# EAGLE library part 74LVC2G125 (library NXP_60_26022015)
Dual bus buffer/line driver; 3-state The 74LVC2G125 provides a dual non-inverting buffer/line driver with 3-state output. The 3-state output is controlled by the output enable input (pin nOE). A HIGH-level at pin nOE causes the output to assume a high-impedance OFF-state. Schmitt trigger action at all inputs makes the circuit highly tolerant of slower input rise and fall times. Inputs can be driven from either 3.3 V or 5 V devices. This feature allows the use of these devices as translators in a mixed 3.3 V and 5 V environment. This device is fully specified for partial power-down applications using IOFF. The IOFF circuitry disables the output, preventing a damaging backflow current through the device when it is powered down. AAL Eindhoven MK
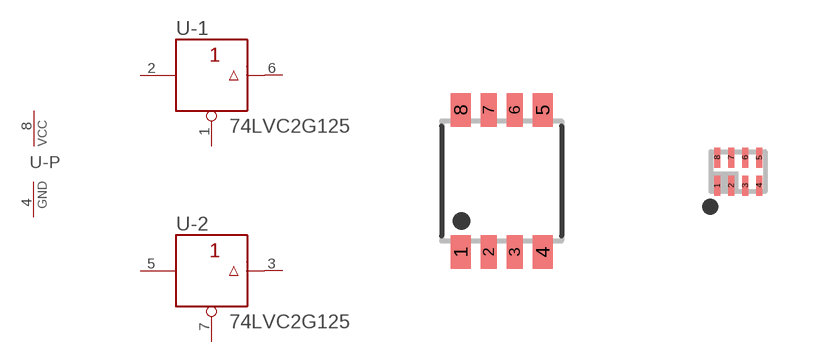
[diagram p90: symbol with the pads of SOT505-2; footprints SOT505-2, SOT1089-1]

Designator prefix U; gates -1=BUFFER_OE -2=BUFFER_OE -P=PWRN

## 74LVC2G125DP  [SOT505-2]
1  -1:!OE  in
2  -1:A  in
3  -2:Y  out
4  -P:GND  pwr
5  -2:A  in
6  -1:Y  out
7  -2:!OE  in
8  -P:VCC  pwr

## 74LVC2G125GF  [SOT1089-1]
Pads as for SOT505-2

## 74LVC2G125GD  [SOT996-2/3]
Pads as for SOT505-2

## 74LVC2G125GM  [SOT902-1/2/3]
1  -2:!OE  in
2  -1:Y  out
3  -2:A  in
4  -P:GND  pwr
5  -2:Y  out
6  -1:A  in
7  -1:!OE  in
8  -P:VCC  pwr

## 74LVC2G125DC  [SOT765]
Pads as for SOT505-2

## 74LVC2G125GT  [SOT833-1]
Pads as for SOT505-2

## Footprint SOT505-2 (pad centres in mm)
SOT505-2 TSSOP8: plastic thin shrink small outline package; 8 leads; body width 3 mm JEDEC: -- IEC: --
smd 0.5 x 0.85: 1 -1.025,-1.775; 4 1.025,-1.775; 5 1.025,1.775; 8 -1.025,1.775
smd 0.4 x 0.85: 2 -0.325,-1.775; 3 0.325,-1.775; 6 0.325,1.775; 7 -0.325,1.775

## Footprint SOT1089-1 (pad centres in mm)
SOT1089-1 XSON8: plastic, extremely thin small outline package; no leads; 8 terminals; body 1 x 1.35 x 0.5 mm JEDEC: -- IEC: -- JEITA: --
smd 0.15 x 0.5: 1 -0.525,-0.35; 2 -0.175,-0.35; 3 0.175,-0.35; 4 0.525,-0.35; 5 0.525,0.35; 6 0.175,0.35; 7 -0.175,0.35; 8 -0.525,0.35

## Footprint SOT996-2/3 (pad centres in mm)
SOT996-2/3 XSON8U: plastic extremely thin small outline package; no leads;8 terminals; UTLP based; body 3 x 2 x 0.5 mm JEDEC: IEC: -- JEITA: --
smd 0.25 x 1.1: 1 -0.75,-1.45
smd 0.25 x 1: 2 -0.25,-1.5; 3 0.25,-1.5; 4 0.75,-1.5; 5 0.75,1.5; 6 0.25,1.5; 7 -0.25,1.5; 8 -0.75,1.5

## Footprint SOT902-1/2/3 (pad centres in mm)
SOT902-1/2/3 XQFN8U: plastic extremely thin quad flat package; no leads; 8 terminals; UTLP based; body 1.6 x 1.6 x 0.5 mm JEDEC: -- IEC: ---
smd 0.4 x 0.32: 1 0.6,-0.55
smd 0.4 x 0.22: 2 0.6,0; 3 0.6,0.5; 5 -0.6,0.5; 6 -0.6,0; 7 -0.6,-0.5
smd 0.22 x 0.4: 4 0,0.6; 8 0,-0.6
